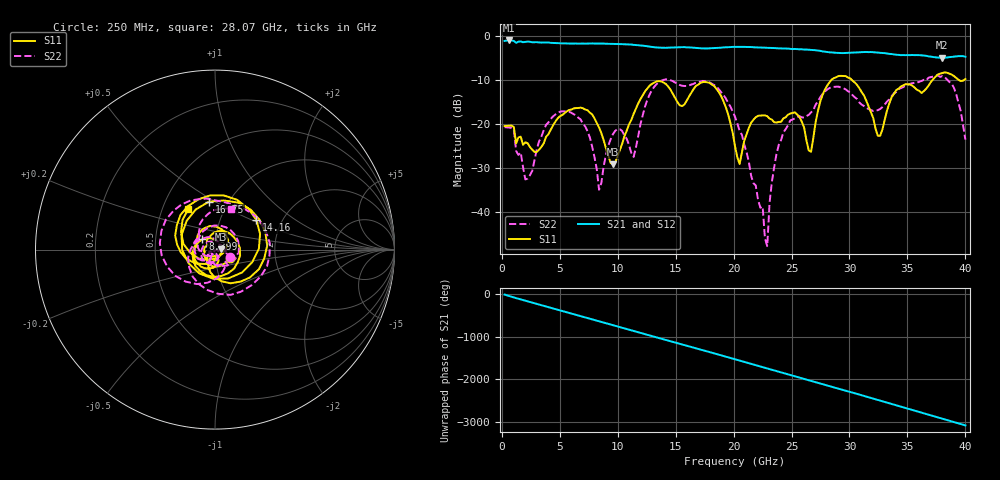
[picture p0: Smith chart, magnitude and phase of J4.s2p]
!Agilent Technologies,E8364B,MY43040528,A.07.50.67
!Agilent E8364B: A.07.50.67
!Date: Thursday, May 22, 2025 22:33:39
!Correction: S11(Full 2 Port(1,2))
!S21(Full 2 Port(1,2))
!S12(Full 2 Port(1,2))
!S22(Full 2 Port(1,2))
!S2P File: Measurements: S11, S21, S12, S22:
# Hz S  dB  R 50
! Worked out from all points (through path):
!   201 points, 250 MHz to 40 GHz, reference 50 ohm
!   highest |S21| = -1.04 dB at 647.5 MHz (marker M1); lowest = -5.0 dB at 38.01 GHz (marker M2)
!   group delay of S21, straight-line fit = 214 ps
!   lowest |S11| = -29.2 dB at 9.591 GHz (marker M3), VSWR 1.07, Z = 53.6 + j0.179 ohm
!   |S11| at or under -10 dB: start of sweep to 28.45 GHz; 30.19 GHz to 37.17 GHz (6.977 GHz wide, 20.7 % of centre); 39.41 GHz to 39.9 GHz (491.4 MHz wide, 1.24 % of centre)
!   |S22| runs from -47.8 to -9.0 dB; largest |S21 - S12| = 0.011
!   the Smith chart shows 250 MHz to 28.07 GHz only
!   S11 on the Smith chart (normalised r, x): 250 MHz: 1.17, -0.11; 8.399 GHz: 0.86, +0.10; 14.16 GHz: 1.48, +0.54; 16.75 GHz: 0.81, +0.47; 28.07 GHz: 0.68, +0.33
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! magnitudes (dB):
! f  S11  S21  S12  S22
! 250 MHz  -20.5  -1.2  -1.1  -20.8
! 647.5 MHz  -20.4  -1.0  -1.0  -20.8
! 2.039 GHz  -24.2  -1.4  -1.4  -32.7
! 4.424 GHz  -20.4  -1.6  -1.6  -18.3
! 7.008 GHz  -16.5  -1.7  -1.7  -20.0
! 8.399 GHz  -20.8  -1.7  -1.7  -35.0
! 9.591 GHz  -29.2  -1.8  -1.8  -22.4
! 11.38 GHz  -17.8  -2.0  -2.0  -27.5
! 13.57 GHz  -10.3  -2.7  -2.7  -10.5
! 14.16 GHz  -10.9  -2.7  -2.7  -9.9
! 16.75 GHz  -11.4  -2.8  -2.7  -10.6
! 18.73 GHz  -12.8  -2.7  -2.7  -12.1
! 20.12 GHz  -25.1  -2.5  -2.5  -18.4
! 22.91 GHz  -18.3  -2.7  -2.7  -47.8
! 23.9 GHz  -19.6  -2.8  -2.8  -24.8
! 26.88 GHz  -23.2  -3.2  -3.2  -16.9
! 28.07 GHz  -11.3  -3.6  -3.6  -12.2
! 30.46 GHz  -10.6  -3.8  -3.7  -14.0
! 32.45 GHz  -22.7  -3.8  -3.8  -16.9
! 33.44 GHz  -15.3  -4.1  -4.0  -14.4
! 38.01 GHz  -8.4  -5.0  -5.0  -9.2
! 40 GHz  -9.8  -4.7  -4.7  -23.6
